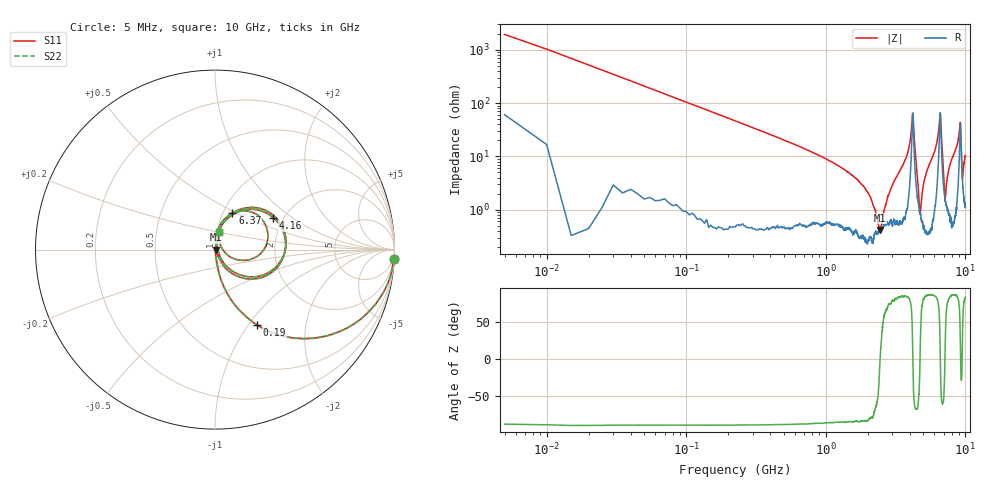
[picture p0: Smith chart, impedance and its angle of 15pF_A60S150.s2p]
! Amotech Co.,Ltd.
! http://www.amotech.co.kr/
! Part Number: A60S150
! These Parameters are Measured in Series Mode Connection
! Operation Temp=25[degC], DC Bias Voltage=0[V]
! Freq. Start=5[MHz] Stop=10[GHz], 2000[Steps]
! Date: Monday, July 13, 2020, 01:37:02
# GHZ S RI R 50.000000
!Freq.(Hz) S11(Real) S11(Imag) S21(Real) S21(Imag) S12(Real) S12(Imag) S22(Real) S22(Imag)
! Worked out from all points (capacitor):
!   2000 points, 5 MHz to 10 GHz, reference 50 ohm
!   read as one part in series: C = 15.3 pF near 55 MHz
!   lowest |Z| = 417 mohm at 2.455 GHz (marker M1)
!   series resonance near 2.449 GHz, so ESL is about 280 pH
!   S11 on the Smith chart (normalised r, x): 5 MHz: 2, -39; 190 MHz: 1.01, -1.10; 4.16 GHz: 1.77, +0.73; 6.37 GHz: 1.11, +0.47; 10 GHz: 1.02, +0.21
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0.005  0.9957 -0.0513  0.00426 0.0513  0.00426 0.0513  0.9957 -0.0513
0.08  0.628 -0.4788  0.372 0.4788  0.372 0.4788  0.628 -0.4788
0.19  0.2331 -0.4189  0.7669 0.4189  0.7669 0.4189  0.2331 -0.4189
0.635  0.0286 -0.1511  0.9714 0.1511  0.9714 0.1511  0.0286 -0.1511
1.675  0.00517 -0.0364  0.9948 0.0364  0.9948 0.0364  0.00517 -0.0364
2.455  0.00415 0.000114  0.9958 -0.000114  0.9958 -0.000114  0.00415 0.000114
2.79  0.00584 0.0169  0.9942 -0.0169  0.9942 -0.0169  0.00584 0.0169
3.34  0.00794 0.0491  0.9921 -0.0491  0.9921 -0.0491  0.00794 0.0491
3.975  0.0475 0.1498  0.9525 -0.1498  0.9525 -0.1498  0.0475 0.1498
4.16  0.3253 0.1775  0.6747 -0.1775  0.6747 -0.1775  0.3253 0.1775
4.275  0.181 -0.163  0.819 0.163  0.819 0.163  0.181 -0.163
4.72  0.00849 -0.00129  0.9915 0.00129  0.9915 0.00129  0.00849 -0.00129
5.005  0.00518 0.0291  0.9948 -0.0291  0.9948 -0.0291  0.00518 0.0291
6.37  0.0969 0.2031  0.9031 -0.2031  0.9031 -0.2031  0.0969 0.2031
6.52  0.2789 0.2197  0.7211 -0.2197  0.7211 -0.2197  0.2789 0.2197
6.67  0.2831 -0.1359  0.7169 0.1359  0.7169 0.1359  0.2831 -0.1359
7.155  0.0149 0.00317  0.9851 -0.00317  0.9851 -0.00317  0.0149 0.00317
7.595  0.0113 0.0546  0.9887 -0.0546  0.9887 -0.0546  0.0113 0.0546
8.335  0.0192 0.1135  0.9808 -0.1135  0.9808 -0.1135  0.0192 0.1135
9.165  0.2766 0.1458  0.7234 -0.1458  0.7234 -0.1458  0.2766 0.1458
9.515  0.035 0.0126  0.965 -0.0126  0.965 -0.0126  0.035 0.0126
10  0.0211 0.1001  0.9789 -0.1001  0.9789 -0.1001  0.0211 0.1001
